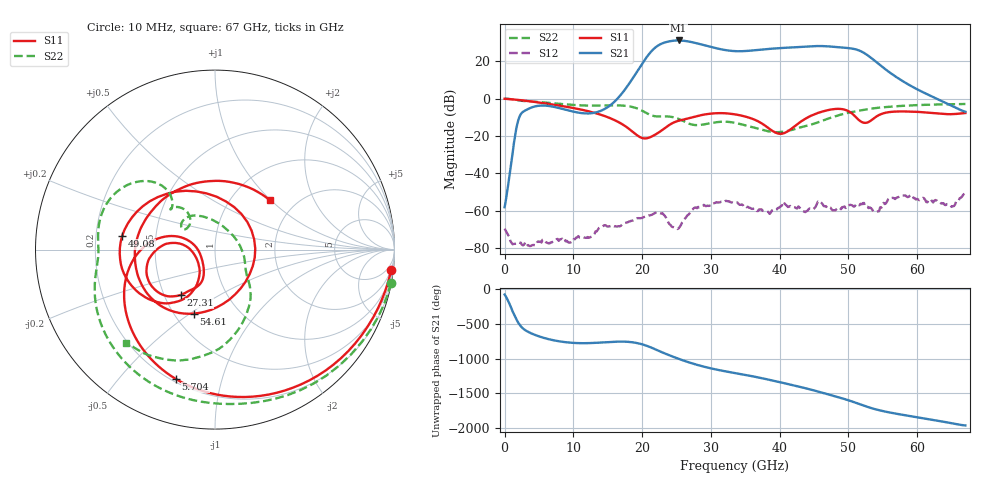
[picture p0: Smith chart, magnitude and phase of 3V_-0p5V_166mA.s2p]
! MARKI MICROWAVE INC.
! Date:  10/23/18
! Model Number:  AMM-6702CH
! Description:  2-port Small Signal S-parameter data for AMM-6702CH
! Frequency Range:  10 MHz to 67 GHz
! Port Configuration:  PORT 1: Input
!  PORT 2: Output
! Bias Condition: Vd = +3V, Vg = -0.5V
! AMM-6702CH s2p files are only valid for small signal conditions (below -5 dBm input power)
!S2P File: Measurements: Mag<S11> Ang<S11>, Mag<S21> Ang<S21>, Mag<S12> Ang<S12>, Mag<S22> Ang<S22>!row 1
# Hz S  dB  R 50
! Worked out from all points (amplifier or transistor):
!   401 points, 10 MHz to 67 GHz, reference 50 ohm
!   highest |S21| = 31.1 dB at 25.3 GHz (marker M1)
!   |S21| within 3 dB of that: 22.21 GHz to 29.5 GHz (7.295 GHz wide, 28.2 % of centre)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
!   unconditionally stable (mu >= 1): start of sweep to end of sweep
!   at 11.06 GHz: K = 2576.37, MAG = -3.9 dB, |S12| = -74.1 dB
!   at 33.51 GHz: K = 13.09, MAG = 26.3 dB, |S12| = -55.5 dB
!   at 67 GHz: K = 152.51, MAG = -3.1 dB, |S12| = -50.5 dB
!   S11 on the Smith chart (normalised r, x): 10 MHz: 2, -17; 5.704 GHz: 0.22, -0.72; 27.31 GHz: 0.61, -0.34; 49.08 GHz: 0.31, +0.07; 54.61 GHz: 0.63, -0.52; 67 GHz: 1.49, +0.99
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1e7  -0.11 -6.7  -58.06 -75.6  -69.50 -157.5  -0.02 -10.8
5.70415e9  -2.46 -106.9  -3.72 20.3  -75.30 137.0  -2.06 -135.0
1.123082e10  -5.96 -165.4  -7.77 -56.3  -74.05 161.6  -3.64 -174.1
1.993952e10  -20.98 -171.8  18.27 -70.6  -63.83 125.9  -6.35 130.6
2.14468e10  -20.18 -134.8  25.65 -124.2  -62.06 118.8  -9.09 132.5
2.245165e10  -18.01 -119.9  28.64 -168.0  -61.03 96.9  -9.56 137.5
2.362398e10  -14.96 -112.5  30.31 142.8  -64.91 56.2  -9.52 136.0
2.529872e10  -11.87 -119.9  31.06 79.0  -69.39 108.5  -10.84 127.7
2.730842e10  -9.98 -127.2  30.10 11.8  -59.41 133.9  -13.93 133.9
2.982055e10  -8.11 -141.8  27.76 -54.8  -57.24 105.3  -13.21 147.4
3.3505e10  -8.43 -170.1  25.36 -126.7  -55.54 42.4  -12.96 122.5
3.718945e10  -12.80 170.6  26.12 164.2  -59.26 -175.8  -16.41 84.6
4.037148e10  -18.75 -147.9  27.05 94.3  -56.90 -4.1  -17.77 29.1
4.238118e10  -14.18 -118.5  27.46 47.9  -58.53 78.6  -16.09 -6.3
4.472582e10  -8.91 -126.1  28.00 -9.9  -58.55 -120.8  -13.73 -33.6
4.707048e10  -6.12 -152.3  27.91 -74.0  -57.86 -148.9  -10.68 -47.9
4.908018e10  -5.63 171.6  27.29 -130.7  -57.97 32.0  -8.39 -61.2
5.058745e10  -8.18 124.1  26.68 -177.8  -57.08 -164.5  -7.12 -70.3
5.209472e10  -12.78 27.6  24.75 129.1  -55.89 141.1  -6.11 -78.5
5.460685e10  -8.52 -108.2  17.87 54.8  -58.09 167.9  -4.80 -92.1
5.594665e10  -7.21 -134.5  14.09 26.4  -53.33 37.7  -4.40 -98.1
6.7e10  -7.72 41.8  -7.04 -161.3  -50.52 -126.7  -2.89 -133.6
